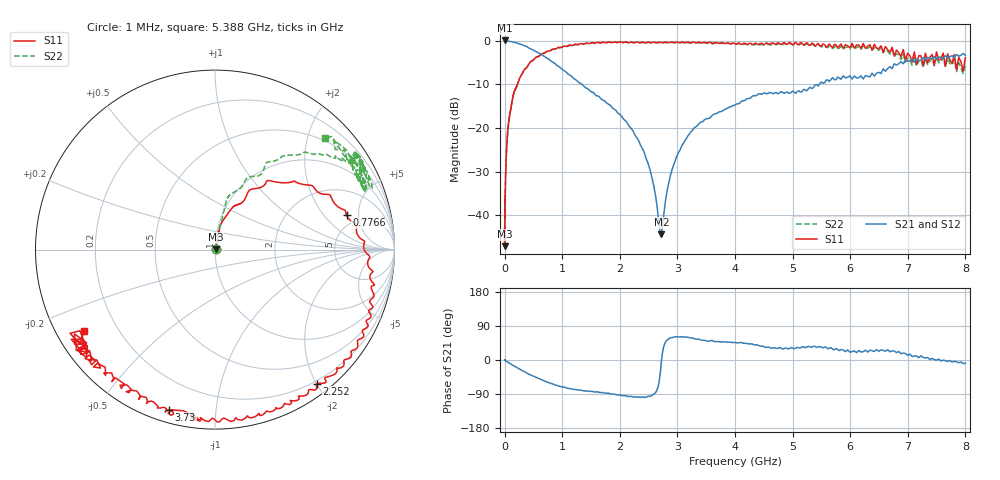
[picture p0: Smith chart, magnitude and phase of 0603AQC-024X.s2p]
!s-Parameter Generated by FASTRON Sdn. Bhd.
!FASTRON P/N : 0603AQC-024X
!Keysight Technologies: E5071C_MY46733604_B.14.02
!Date: Thu Jun 25 13:52:43 2026
!Version  :Rev00  Thu Jun 25 13:52:43 2026
!Data & Calibration Information:
!Freq  S11:SOLT2(ON)  S21:SOLT2(ON)  S12:SOLT2(ON)  S22:SOLT2(ON)
!PortZ  Port1:50+j0  Port2:50+j0
!When reading reference impedance value at option line is always used.
! Remarks : This data is being provided solely for informational purposes.
# Hz S dB R 50
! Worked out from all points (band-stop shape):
!   1601 points, 1 MHz to 8 GHz, reference 50 ohm
!   highest |S21| = 0.02 dB at 7.138 MHz (marker M1); lowest = -44.4 dB at 2.722 GHz (marker M2)
!   |S21| within 3 dB of the highest: start of sweep to 610.7 MHz; 7.958343 GHz to 7.964345 GHz (6.002 MHz wide, 0.0754 % of centre)
!   lowest |S11| = -47.1 dB at 1.541 MHz (marker M3), VSWR 1.01, Z = 50.4 + j0.173 ohm
!   |S11| at or under -10 dB: start of sweep to 223.6 MHz
!   |S22| runs from -45.9 to -0.4 dB; largest |S21 - S12| = 0.013
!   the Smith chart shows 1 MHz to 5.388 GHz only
!   S11 on the Smith chart (normalised r, x): 1 MHz: 1.01, +0.00; 776.6 MHz: 3.93, +3.55; 2.252 GHz: 0.16, -2.00; 3.73 GHz: 0.06, -0.75; 5.388 GHz: 0.08, -0.29
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1000000  -44.50 11.9  -0.06 -0.2  -0.05 -0.1  -44.00 16.7
1541011  -47.10 22.8  -0.06 -0.3  -0.06 -0.2  -45.00 7.9
4479405  -41.00 50.8  -0.05 -0.5  -0.05 -0.5  -41.00 57.1
7138274  -37.30 55.8  0.02 -0.9  -0.02 -0.7  -37.50 61.5
2.00676e7  -30.10 71.6  -0.07 -2.1  -0.08 -2.0  -29.80 79.7
8.994653e7  -17.00 77.5  -0.18 -8.9  -0.18 -8.8  -17.10 77.3
2.123148e8  -10.40 60.2  -0.55 -19.8  -0.55 -19.8  -10.40 76.0
4.006501e8  -5.92 48.2  -1.50 -35.8  -1.50 -35.9  -5.80 58.5
7.765934e8  -2.41 14.7  -4.37 -60.5  -4.36 -60.6  -2.35 44.2
1.171668e9  -1.15 -9.5  -8.33 -77.0  -8.33 -77.2  -1.07 33.2
1.7949e9  -0.39 -33.7  -14.50 -87.7  -14.60 -87.9  -0.41 34.0
2.252141e9  -0.55 -52.8  -21.30 -97.9  -21.30 -98.1  -0.42 28.9
2.44288e9  -0.54 -60.3  -26.40 -98.4  -26.40 -98.4  -0.47 28.9
2.63362e9  -0.53 -65.6  -36.60 -83.2  -36.60 -83.2  -0.48 31.3
2.721653e9  -0.47 -68.9  -44.40 -5.2  -44.20 -5.2  -0.48 33.5
3.061592e9  -0.42 -79.6  -24.60 61.6  -24.60 61.6  -0.46 33.7
3.730463e9  -0.65 -106.0  -16.30 48.1  -16.30 47.9  -0.62 27.8
4.744521e9  -0.49 -140.0  -12.20 30.6  -12.10 30.3  -0.80 21.9
5.388334e9  -1.30 -148.0  -10.20 36.1  -10.10 35.8  -1.21 45.4
6.419251e9  -0.86 -174.0  -8.17 22.7  -8.15 22.3  -1.61 44.8
7.306013e9  -2.87 153.0  -4.41 5.3  -4.41 4.5  -4.14 39.7
8e9  -3.93 141.0  -3.41 -8.4  -3.44 -9.2  -5.46 48.7
